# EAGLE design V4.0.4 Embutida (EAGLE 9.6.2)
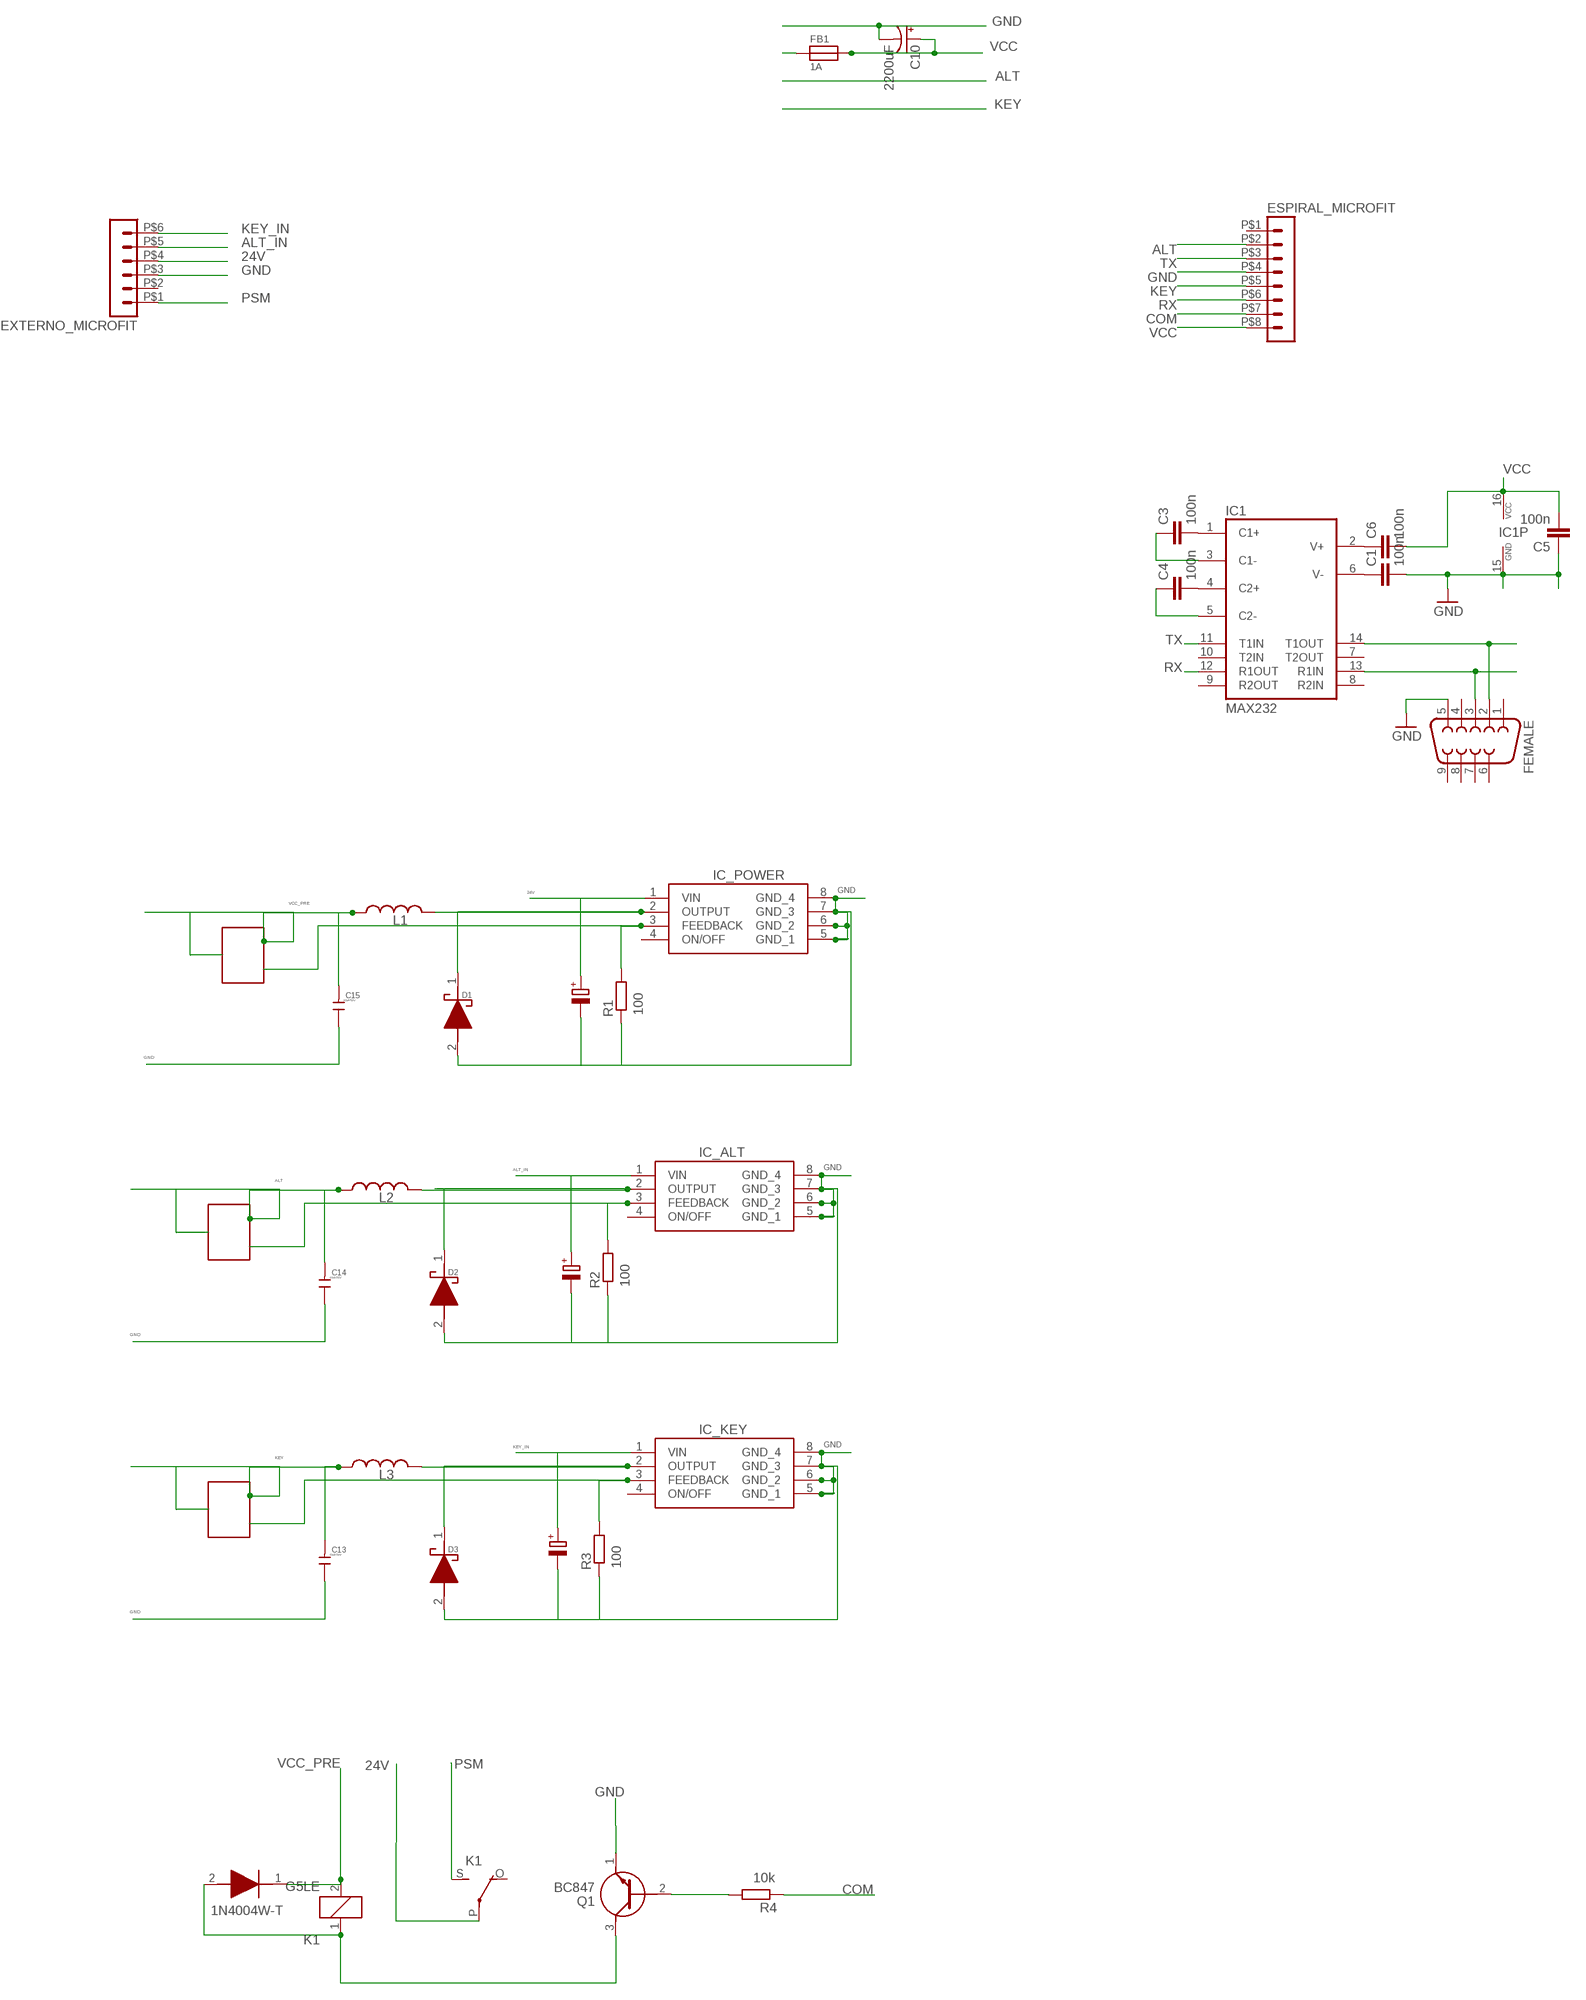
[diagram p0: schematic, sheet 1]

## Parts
C1  100n  C-EUC0805  [C0805]
C2  22uF/50v  CPOL-EUD  [PANASONIC_D]
C3  100n  C-EUC0805  [C0805]
C4  100n  C-EUC0805  [C0805]
C5  100n  C-EUC0805  [C0805]
C6  100n  C-EUC0805  [C0805]
C8  22uF/50V  CPOL-EUD  [PANASONIC_D]
C9  22uF/50V  CPOL-EUD  [PANASONIC_D]
C10  2200uF  CAP_POL  [PANASONIC_H13_MOD]
C13  10uF/50V  C-0805  [C0805]
C14  10uF/50V  C-0805  [C0805]
C15  10uF/50V  C-0805  [C0805]
D1  1N5819HW1-7-F  [SODFL3518X115N]
D2  1N5819HW1-7-F  [SODFL3518X115N]
D3  1N5819HW1-7-F  [SODFL3518X115N]
D5  1N4004W-T  [SODFL3818X130N]
ESPIRAL_MICROFIT  HEADER_POS8_43045-0800  [43045-0800]
EXTERNO_MICROFIT  HEADER_POS6_43045-0600  [43045-0600]
FB1  1A  FERRITE0805  [0805]
FEMALE  F09H  [F09H]
IC1  MAX232  MAX232ECWES  [SO16]
IC_ALT  XL1509-3.3E1  [SOIC127P600X175-8N]
IC_KEY  XL1509-3.3E1  [SOIC127P600X175-8N]
IC_POWER  XL1509-3.3E1  [SOIC127P600X175-8N]
K1  G5LE  [G5LE]
L1  47uH  INDUCTOR  [SDE0604A-470M]
L2  47uH  INDUCTOR  [SDE0604A-470M]
L3  47uH  INDUCTOR  [SDE0604A-470M]
Q1  BC847  [BC847]
R1  100  R-EU_R0805  [R0805]
R2  100  R-EU_R0805  [R0805]
R3  100  R-EU_R0805  [R0805]
R4  10k  R-EU_R0805  [R0805]
T1  TRIMPOT 10K  TRIMPOT  [TRIMPOT]
T2  TRIMPOT 10K  TRIMPOT  [TRIMPOT]
T3  TRIMPOT 10K  TRIMPOT  [TRIMPOT]

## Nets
24V: C2.+ EXTERNO_MICROFIT.P$4 IC_POWER.1(VIN) K1.P(2:P)
ALT: C14.2 ESPIRAL_MICROFIT.P$2 L2.1 T2.VCC1 T2.VCC2
ALT_IN: C8.+ EXTERNO_MICROFIT.P$5 IC_ALT.1(VIN)
COM: ESPIRAL_MICROFIT.P$7 R4.1
GND: C1.2 C2.- C5.1 C8.- C9.- C10.- C13.1 C14.1 C15.1 D1.2(A) D2.2(A) D3.2(A) ESPIRAL_MICROFIT.P$4 EXTERNO_MICROFIT.P$3 FEMALE.5 IC1.15(GND) IC_ALT.5(GND_1) IC_ALT.6(GND_2) IC_ALT.7(GND_3) IC_ALT.8(GND_4) IC_KEY.5(GND_1) IC_KEY.6(GND_2) IC_KEY.7(GND_3) IC_KEY.8(GND_4) IC_POWER.5(GND_1) IC_POWER.6(GND_2) IC_POWER.7(GND_3) IC_POWER.8(GND_4) Q1.1(E) R1.1 R2.1 R3.1
KEY: C13.2 ESPIRAL_MICROFIT.P$5 L3.1 T3.VCC1 T3.VCC2
KEY_IN: C9.+ EXTERNO_MICROFIT.P$6 IC_KEY.1(VIN)
N$1: D1.1(K) IC_POWER.2(OUTPUT) L1.2
N$2: D2.1(K) IC_ALT.2(OUTPUT) L2.2
N$4: IC_ALT.3(FEEDBACK) R2.2 T2.OUT
N$5: D3.1(K) IC_KEY.2(OUTPUT) L3.2
N$6: IC_KEY.3(FEEDBACK) R3.2 T3.OUT
N$7: D5.2(A) K1.1 Q1.3(C)
N$8: IC_POWER.3(FEEDBACK) R1.2 T1.OUT
N$10: Q1.2(B) R4.2
N$11: C3.2 IC1.1(C1+)
N$12: C4.2 IC1.4(C2+)
N$13: C3.1 IC1.3(C1-)
N$17: C4.1 IC1.5(C2-)
N$18: C6.1 IC1.2(V+)
N$19: C1.1 IC1.6(V-)
N$20: FEMALE.2 IC1.14(T1OUT)
N$30: FEMALE.3 IC1.13(R1IN)
PSM: EXTERNO_MICROFIT.P$1 K1.S(2:S)
RX: ESPIRAL_MICROFIT.P$6 IC1.12(R1OUT)
TX: ESPIRAL_MICROFIT.P$3 IC1.11(T1IN)
VCC: C5.2 C6.2 C10.+ ESPIRAL_MICROFIT.P$8 FB1.2 IC1.16(VCC)
VCC_PRE: C15.2 D5.1(K) FB1.1 K1.2 L1.1 T1.VCC1 T1.VCC2
Unconnected: ESPIRAL_MICROFIT.P$1 EXTERNO_MICROFIT.P$2 FEMALE.1 FEMALE.4 FEMALE.6 FEMALE.7 FEMALE.8 FEMALE.9 IC1.7(T2OUT) IC1.8(R2IN) IC1.9(R2OUT) IC1.10(T2IN) IC_ALT.4(ON/OFF) IC_KEY.4(ON/OFF) IC_POWER.4(ON/OFF) K1.O(2:O)

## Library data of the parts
C1 C3-C6 = rcl@1:C-EU: CAPACITOR, European symbol; MPN: C0805C104K8RACAUTO
C2 C8 C9 = rcl:CPOL-EU: POLARIZED CAPACITOR, European symbol; MPN: EEH-ZA1H220P; SPICEPREFIX: C
C10 = SparkFun-Capacitors:CAP_POL: Capacitor Polarized; MPN: EEV-FK1A222Q
C13-C15 = discrete:C*: Ceramic Capacitors; MPN: C2012X5R1H106K125AC
D1-D3 = 1N5819HW1-7-F:1N5819HW1-7-F: 1N5819 Schottky Diode 40V 1A SOD123F; ARROW_PART_NUMBER: 1N5819HW1-7-F; ARROW_PRICE-STOCK: https://www.arrow.com/en/products/1n5819hw1-7-f/diodes-incorporated?region=nac; DESCRIPTION: 1N5819 Schottky Diode 40V 1A SOD123F; HEIGHT: 1.15mm; MANUFACTURER_NAME: Diodes Inc.; MANUFACTURER_PART_NUMBER: 1N5819HW1-7-F; MOUSER_PART_NUMBER: 621-1N5819HW1-7-F; MOUSER_PRICE-STOCK: https://www.mouser.co.uk/ProductDetail/Diodes-Incorporated/1N5819HW1-7-F?qs=60RJRzIpcl9ACQG7Zn63jQ%3D%3D; MPN: 1N5822 SS34
D5 = 1N4004W-T:1N4004W-T: Rectifiers SOD-123,1A,400V,GP; DESCRIPTION: Rectifiers SOD-123,1A,400V,GP; HEIGHT: 1.3mm; MANUFACTURER_NAME: Rectron; MANUFACTURER_PART_NUMBER: 1N4004W-T; MOUSER_PART_NUMBER: 583-1N4004W-T; MOUSER_PRICE-STOCK: https://www.mouser.co.uk/ProductDetail/Rectron/1N4004W-T?qs=QNEnbhJQKvYW6o2Wv4Vvaw%3D%3D
ESPIRAL_MICROFIT = con-molex-micro-fit-3_0 (1):HEADER_POS8_?: Molex - Micro-Fit 3.0 Series connector, 3.00mm (0.118") pitch header, 8 positions.; MPN: 43045-0800
EXTERNO_MICROFIT = con-molex-micro-fit-3_0 (1):HEADER_POS6_?: Molex - Micro-Fit 3.0 Series connector, 3.00mm (0.118") pitch header, 6 positions.; MPN: 43045-0600
FB1 = microbuilder:FERRITE: Ferrite Bead; MPN: BLM21AG121SN1D
FEMALE = con-subd:F09: SUB-D; MPN: FEMALE DR9; OC_FARNELL: unknown; OC_NEWARK: unknown
IC1 = maxim-6b:MAX232ECWE: RS232 TRANSEIVER; MPN: MAX3232CSE+
IC_ALT IC_KEY IC_POWER = XL1509-3.3E1:XL1509-3.3E1: 40V 2A SOP-8_150mil DC-DC Converters RoHS Source: Datasheet; DESCRIPTION: 40V 2A SOP-8_150mil DC-DC Converters RoHS; HEIGHT: 1.75mm; MANUFACTURER_NAME: XLSEMI; MANUFACTURER_PART_NUMBER: XL1509-3.3E1; MPN: XL1509-ADJE1
K1 = relay:G5LE: RELAY 1 x switch, 10 A/120 V AC, 8 A/30 V DC, Omron
L1-L3 = passives:INDUCTOR: A very specific inductor; MPN: SDE0604A-470M
Q1 = BC847:BC847: Epitaxial Planar NPN transistor Source: Datasheet; DESCRIPTION: Epitaxial Planar NPN transistor; HEIGHT: 1.3mm; MANUFACTURER_NAME: KEC; MANUFACTURER_PART_NUMBER: BC847
R1-R4 = rcl:R-EU_: RESISTOR, European symbol; MPN: RA73F2A100RBTDF; SPICEPREFIX: R
T1-T3 = TRIMPOT:TRIMPOT; MPN: EVM3ESX50B14

## Module LDR
Ports: 

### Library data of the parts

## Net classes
1 New Class: width 0.5 mm, drill 1 mm

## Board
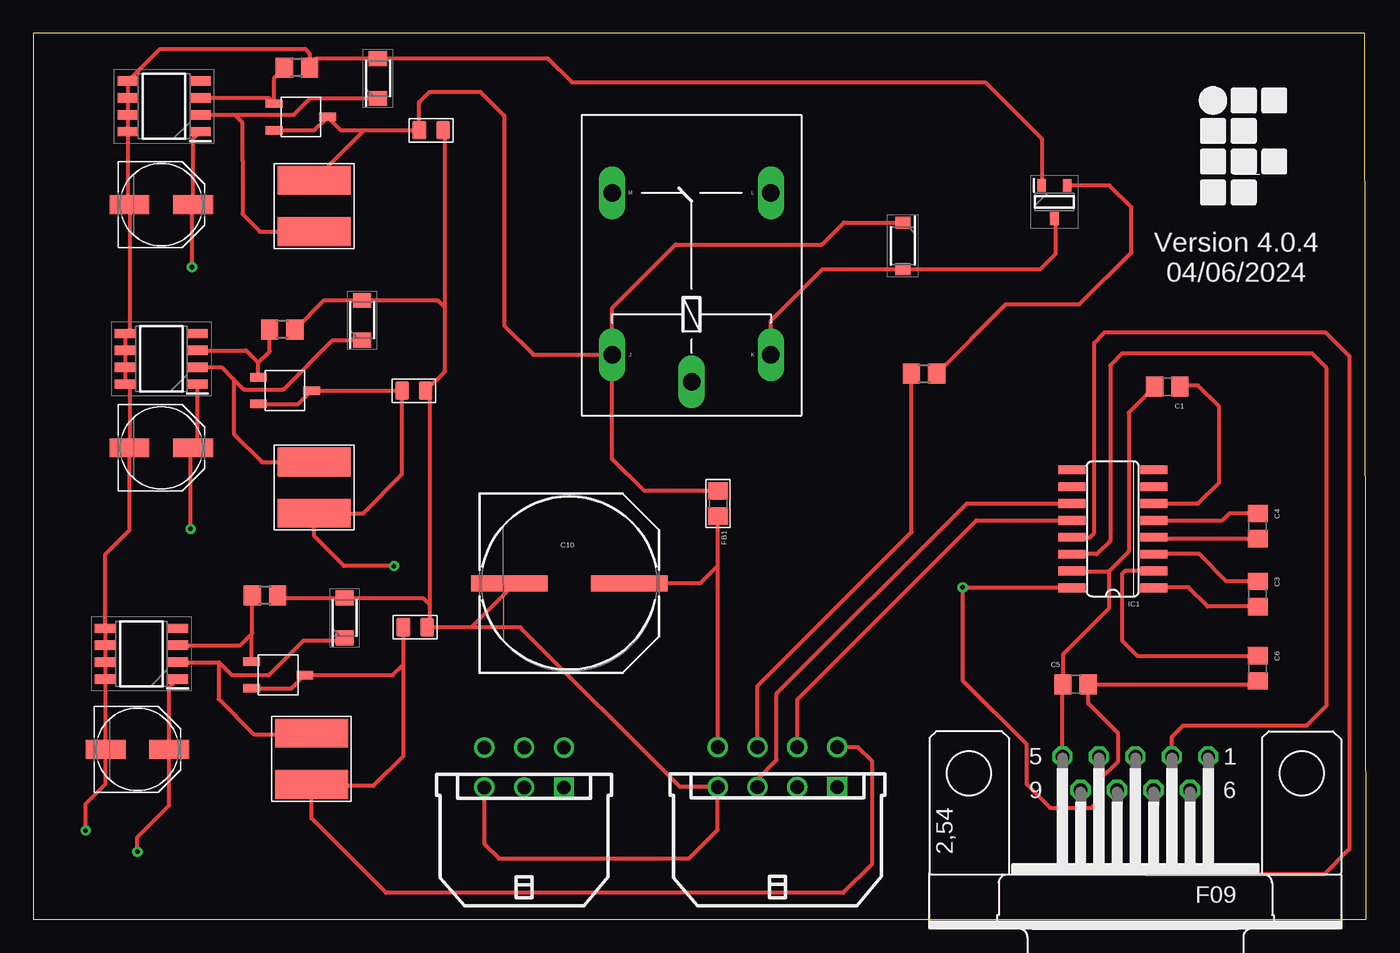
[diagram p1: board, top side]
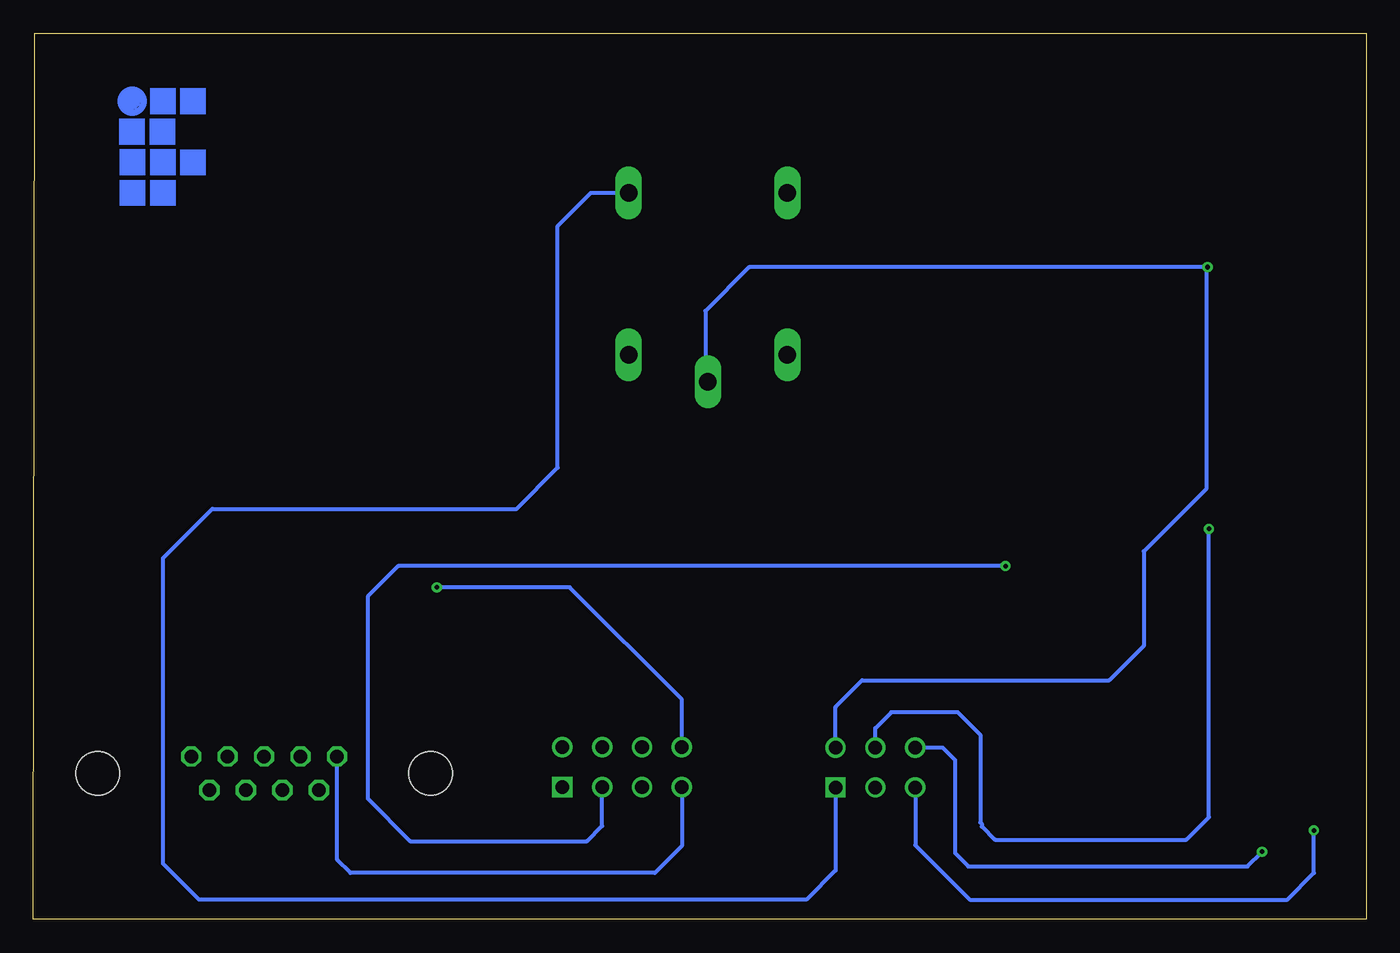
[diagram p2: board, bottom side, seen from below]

Size 100.32 x 66.7 mm. Coordinates in mm from the lower left corner, seen from the top.
Outline: 0,0 100.32,0 100.2,66.7 0,66.7 0,0
Copper layers (1*16): Top 0.035mm / dielectric 1.5mm / Bottom 0.035mm
Design rules "default *": minimum track width 6mil, minimum drill 0.35mm, track to track 6mil, track to pad 6mil, pad to pad 6mil, via to via 6mil, smd to smd 6mil, copper to edge 40mil, drill to drill 6mil, minimum pad ring 10mil, minimum via ring 8mil, stop-mask expansion 4mil, vias tented up to drill 0mil, thermal gap 10mil

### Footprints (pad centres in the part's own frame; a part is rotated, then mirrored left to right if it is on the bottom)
C0805 = smd 1.3 x 1.5: 1 -0.95,0; 2 0.95,0
PANASONIC_D = smd 3 x 1.4: + 2.4,0; - -2.4,0
PANASONIC_H13_MOD = smd 5.75 x 1.2: + 4.5,0; - -4.5,0
C0805' = smd 1.016 x 1.397: 1 -0.889,0; 2 0.889,0
SODFL3518X115N = smd 1.12 x 1.37: 1 -1.5,0; 2 1.5,0
SODFL3818X130N = smd 0.92 x 1.13: 1 -1.75,0; 2 1.75,0
43045-0800 = drill 1.02 square: P$1 4.5,4.32 | drill 1.02: P$2 1.5,4.32; P$3 -1.5,4.32; P$4 -4.5,4.32; P$5 4.5,7.32; P$6 1.5,7.32; P$7 -1.5,7.32; P$8 -4.5,7.32
43045-0600 = drill 1.02 square: P$1 3,4.32 | drill 1.02: P$2 0,4.32; P$3 -3,4.32; P$4 3,7.32; P$5 0,7.32; P$6 -3,7.32
0805 = smd 1.3 x 1.5: 1 -0.95,0; 2 0.95,0
F09H = drill 1.016 octagon: 1 -5.486,-1.27; 2 -2.743,-1.27; 3 0,-1.27; 4 2.743,-1.27; 5 5.486,-1.27; 6 -4.115,1.27; 7 -1.372,1.27; 8 1.372,1.27; 9 4.115,1.27 | hole 3.302: -12.522,0; 12.522,0
SO16 = smd 0.66 x 2.032: 1 -4.445,-3.073; 2 -3.175,-3.073; 3 -1.905,-3.073; 4 -0.635,-3.073; 5 0.635,-3.073; 6 1.905,-3.073; 7 3.175,-3.073; 8 4.445,-3.073; 9 4.445,3.073; 10 3.175,3.073; 11 1.905,3.073; 12 0.635,3.073; 13 -0.635,3.073; 14 -1.905,3.073; 15 -3.175,3.073; 16 -4.445,3.073
SOIC127P600X175-8N = smd 1.55 x 0.7: 1 -2.725,1.905; 2 -2.725,0.635; 3 -2.725,-0.635; 4 -2.725,-1.905; 5 2.725,-1.905; 6 2.725,-0.635; 7 2.725,0.635; 8 2.725,1.905
G5LE = drill 1.321 long: 1 -7.493,-5.969; 2 -7.493,5.969; O 4.699,5.969; P -9.525,0; S 4.699,-5.969
SDE0604A-470M = smd 2.15 x 5.5: 1 -1.931,0; 2 1.931,0
BC847 = smd 0.95 x 0.65: 1 -1.25,-0.95; 2 -1.25,0.95; 3 1.25,0
R0805 = smd 1.3 x 1.5: 1 -0.95,0; 2 0.95,0
TRIMPOT = smd 1.27 x 0.635: OUT 0.5,0.5; VCC1 -3.5,1.5; VCC2 0.5,2.5

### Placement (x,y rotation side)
C1  85.34,40.09 180 top
C2  9.64,53.79 0 top
C3  92.14,24.49 270 top
C4  92.14,29.59 270 top
C5  78.44,17.69 0 top
C6  92.14,18.89 270 top
C8  9.64,35.49 0 top
C9  7.84,12.79 0 top
C10  40.34,25.29 0 top
C13  10uF/50V  [C0805']  28.74,21.99 180 top
C14  10uF/50V  [C0805']  28.64,39.79 180 top
C15  10uF/50V  [C0805']  29.94,59.39 180 top
D1  25.94,63.29 90 top
D2  24.74,45.09 90 top
D3  23.44,22.69 90 top
D5  65.44,50.69 270 top
ESPIRAL_MICROFIT  56.01,5.64 0 top
EXTERNO_MICROFIT  36.94,5.62 0 top
FB1  51.54,31.29 270 top
FEMALE  82.94,10.99 180 top
IC1  81.24,29.39 90 top
IC_ALT  9.64,42.19 180 top
IC_KEY  8.14,19.99 180 top
IC_POWER  9.84,61.19 180 top
K1  49.54,49.99 90 top
L1  21.14,53.69 270 top
L2  21.14,32.49 90 top
L3  20.94,12.09 90 top
Q1  76.84,53.99 270 top
R1  19.84,64.09 180 top
R2  18.74,44.39 180 top
R3  17.44,24.39 180 top
R4  67.04,41.09 0 top
T1  18.64,61.89 180 top
T2  17.44,41.29 180 top
T3  16.94,19.89 180 top

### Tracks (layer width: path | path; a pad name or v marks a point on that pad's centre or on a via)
24V  (via drill 0.35)
  Top 0.305: IC_POWER.1 12.04,58.76 C2.+ 11.94,53.69 v11.94,49.09
  Bottom 0.305: EXTERNO_MICROFIT.P$4 39.94,15.99 37.94,17.99 19.34,17.99 16.74,20.59 16.74,27.69 12.04,32.39 12.04,48.99 v11.94,49.09 46.44,49.09 49.74,45.79 49.74,40.67 K1.P
ALT  (via drill 0.35)
  Top 0.305: T2.VCC2 19.94,38.79 T2.VCC1 C14.2 27.75,33.51 24.81,30.56 L2.1 21.14,28.84 23.39,26.59 v27.14,26.59
  Bottom 0.305: v27.14,26.59 72.84,26.59 75.14,24.29 75.14,9.09 71.94,5.89 58.64,5.89 57.51,7.03 ESPIRAL_MICROFIT.P$2
ALT_IN  (via drill 0.35)
  Top 0.305: IC_ALT.1 12.37,35.82 C8.+ 11.84,35.29 v11.84,29.39
  Bottom 0.305: EXTERNO_MICROFIT.P$5 36.94,14.39 35.74,15.59 30.74,15.59 29.04,13.89 29.04,7.29 28.94,7.19 28.94,6.99 27.94,5.99 13.54,5.99 11.84,7.69 v11.84,29.39
COM
  Top 0.305: ESPIRAL_MICROFIT.P$7 54.51,17.56 66.09,29.14 R4.1
GND  (via drill 0.35)
  Top 0.305: C1.2 82.44,38.14 82.44,27.69 80.94,26.19 | IC1.15 78.2,26.19 80.94,26.19 | 80.94,26.19 80.94,23.39 77.49,19.94 77.49,17.99 | 77.49,17.99 C5.1 | FEMALE.5 77.46,17.96 77.49,17.99 | 29.83,23.69 29.83,39.49 C14.1 30.94,41.21 30.94,46.09 | 29.83,23.69 29.83,22.19 C13.1 32.94,21.99 | 30.94,46.09 30.94,59.28 C15.1 | Q1.1 75.89,58.74 71.64,62.99 40.54,62.99 38.74,64.79 D1.2 21.29,64.79 20.79,64.29 R1.1 20.79,65.19 20.46,65.53 9.55,65.53 IC_POWER.5 IC_POWER.6 IC_POWER.7 IC_POWER.8 7.12,53.92 C2.- 7.24,44.42 IC_ALT.5 IC_ALT.6 IC_ALT.7 IC_ALT.8 7.24,39.96 C8.- 7.24,29.29 5.42,27.47 IC_KEY.5 IC_KEY.6 IC_KEY.7 IC_KEY.8 5.42,12.82 C9.- 5.44,10.19 3.94,8.69 v3.94,6.69 | R2.1 21.89,46.59 D2.2 30.44,46.59 30.94,46.09 | EXTERNO_MICROFIT.P$3 33.94,5.69 35.04,4.59 49.34,4.59 51.51,6.76 ESPIRAL_MICROFIT.P$4 48.68,9.96 36.69,21.94 36.69,21.99 32.94,21.99 | R3.1 18.59,24.19 D3.2 29.33,24.19 29.83,23.69 | 32.94,21.99 35.64,24.69 C10.-
  Bottom 0.305: ESPIRAL_MICROFIT.P$4 51.51,5.53 53.54,3.49 76.44,3.49 77.44,4.49 77.44,12.25 FEMALE.5 | EXTERNO_MICROFIT.P$3 33.94,5.59 29.84,1.49 5.94,1.49 3.94,3.49 v3.94,6.69
KEY
  Top 0.305: ESPIRAL_MICROFIT.P$5 62.08,12.96 63.14,11.89 63.14,4.19 60.94,1.99 26.54,1.99 20.94,7.59 L3.1 21.06,10.04 25.59,10.04 27.85,12.31 27.85,19.19 | T3.VCC2 19.44,17.39 T3.VCC1 27.05,18.39 27.85,19.19 | 27.85,19.19 C13.2
KEY_IN  (via drill 0.35)
  Top 0.305: v7.84,5.09 7.84,6.19 10.24,8.59 C9.+ 10.24,17.46 IC_KEY.1
  Bottom 0.305: EXTERNO_MICROFIT.P$6 31.89,12.94 30.94,11.99 30.94,4.99 29.94,3.99 8.94,3.99 v7.84,5.09
N$1
  Top 0.305: IC_POWER.2 15.14,60.56 | 15.14,60.56 19.61,60.56 20.84,61.79 D1.1 | 15.14,60.56 15.74,59.96 15.74,57.29 15.74,57.09 15.74,53.09 17.07,51.76 L1.2
N$2
  Top 0.305: IC_ALT.2 14.18,41.56 15.09,40.64 | 15.09,40.64 15.84,39.89 18.84,39.89 22.54,43.59 D2.1 | 15.09,40.64 15.09,36.54 17.21,34.43 L2.2
N$4
  Top 0.305: T2.OUT 16.94,41.89 | IC_ALT.3 16.01,42.83 16.94,41.89 | R2.2 17.79,42.74 16.94,41.89
N$5
  Top 0.305: D3.1 23.44,20.99 20.34,20.99 17.74,18.39 14.94,18.39 13.98,19.36 | IC_KEY.2 13.98,19.36 | 13.98,19.36 13.94,19.32 13.94,16.59 16.59,13.94 20.86,13.94 L3.2
N$6
  Top 0.305: T3.OUT 16.44,21.49 | IC_KEY.3 15.58,20.63 16.44,21.49 | 16.44,21.49 16.49,21.54 R3.2
N$7
  Top 0.305: K1.1 55.51,45.06 59.39,48.94 D5.2 75.79,48.94 76.94,50.09 76.94,52.64 Q1.3
N$8
  Top 0.305: IC_POWER.3 17.71,61.83 T1.OUT 18.14,63.34 R1.2
N$10
  Top 0.305: R4.2 73.19,46.29 78.74,46.29 82.64,50.19 82.64,53.59 80.99,55.24 Q1.2
N$11
  Top 0.305: C3.2 88.39,23.54 86.94,24.99 84.36,24.99 IC1.1
N$12
  Top 0.305: C4.2 84.43,28.64 IC1.4
N$13
  Top 0.305: C3.1 89.79,25.44 87.75,27.49 IC1.3
N$17
  Top 0.305: C4.1 89.99,30.54 89.44,29.99 84.35,29.99 IC1.5
N$18
  Top 0.305: IC1.2 82.17,26.22 81.94,25.99 81.94,20.99 83.09,19.84 C6.1
N$19
  Top 0.305: IC1.6 87.65,31.3 89.24,32.89 89.24,38.59 87.64,40.19 86.39,40.19 C1.1
N$20
  Top 0.305: FEMALE.2 85.69,13.74 86.54,14.59 95.84,14.59 97.34,16.09 97.34,41.49 96.24,42.59 81.94,42.59 81.04,41.69 81.04,28.49 80.04,27.49 IC1.14
N$30
  Top 0.305: IC1.13 79.51,28.76 79.84,29.09 79.84,43.39 80.64,44.19 97.24,44.19 99.07,42.36 99.07,5.33 99.03,5.28 98.97,5.23 97.14,3.39 83.74,3.39 82.94,4.19 FEMALE.3
PSM
  Bottom 0.305: EXTERNO_MICROFIT.P$1 39.94,3.69 42.14,1.49 87.84,1.49 90.54,4.19 90.54,27.19 86.84,30.89 63.94,30.89 60.84,33.99 60.84,52.19 58.34,54.69 K1.S
RX
  Top 0.305: ESPIRAL_MICROFIT.P$6 57.51,16.56 70.98,30.03 IC1.12
TX
  Top 0.305: ESPIRAL_MICROFIT.P$3 54.51,10.56 55.94,11.99 55.94,16.99 70.25,31.3 IC1.11
VCC  (via drill 0.35)
  Top 0.305: 51.51,30.19 51.51,26.59 | 51.51,26.59 ESPIRAL_MICROFIT.P$8 | 51.51,30.19 51.51,30.31 | 51.51,30.31 FB1.2 | 51.47,30.34 51.51,30.31 | IC1.16 78.13,24.99 v69.94,24.99 69.94,17.99 74.74,13.19 74.74,10.19 76.54,8.39 79.64,8.39 80.24,8.99 80.24,10.49 81.64,11.89 81.64,13.99 79.39,16.24 C5.2 | 91.69,17.49 91.89,17.69 | C5.2 91.89,17.69 | 91.89,17.69 C6.2 | 79.44,17.64 C5.2 | 51.41,30.29 51.51,30.19 | 51.51,26.59 50.22,25.31 50.21,25.29 C10.+
  Bottom 0.305: ESPIRAL_MICROFIT.P$8 51.51,16.56 59.94,24.99 v69.94,24.99
VCC_PRE
  Top 0.305: T1.VCC2 21.14,59.39 T1.VCC1 23.14,59.39 24.91,59.39 | K1.2 43.57,46.03 48.34,50.79 59.34,50.79 60.99,52.44 D5.1 | FB1.1 45.99,32.24 43.57,34.66 K1.2 | K1.2 37.64,42.5 35.44,44.69 35.44,60.49 33.64,62.29 29.84,62.29 29.05,61.51 C15.2 24.91,59.39 | L1.1 24.91,59.39
(copper drawn outside any net)
  shapes: Bottom area x9, Bottom circle x3

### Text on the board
tNames: M | L | Version 4.0.4 / 04/06/2024 | J | K

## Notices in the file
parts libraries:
SparkFun-Capacitors: Licensing: CC v3.0 Share-Alike You are welcome to use this library for commercial purposes.
